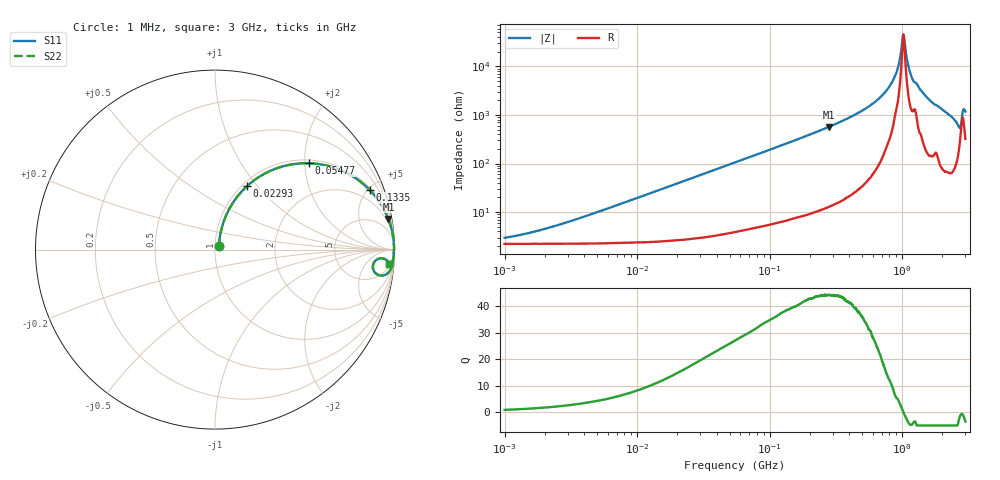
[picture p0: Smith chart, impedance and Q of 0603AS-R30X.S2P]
!s-Parameter Generated by FASTRON Sdn. Bhd.
!FASTRON P/N : 0603AS-R30X
!Keysight Technologies: E4991B_MY54100416_A.01.15
!Date created: Tue Oct 17 15:01:34 2023
!Version  : Rev01 Tue Oct 17 15:01:34 2023
!Data & Calibration Information:
!Freq	S11	S21	S12	S22
!PortZ  Port1:50+j0  Port2:50+j0
!When reading reference impedance value at option line is always used.
! Remarks : This data is being provided solely for informational purposes.
# Hz S dB R 50
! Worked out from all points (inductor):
!   1601 points, 1 MHz to 3 GHz, reference 50 ohm
!   read as one part in series: L = 309 nH near 3.459 MHz
!   highest Q = 44.3 at 278.5 MHz (marker M1), where L = 323 nH
!   self-resonance near 1.018 GHz
!   S11 on the Smith chart (normalised r, x): 1 MHz: 1.04, +0.04; 22.93 MHz: 1.05, +0.89; 54.77 MHz: 1.08, +2.10; 133.5 MHz: 1.13, +5.14; 3 GHz: 7, -23
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1000000  -30.77 40.4  -0.19 -1.1  -0.19 -1.1  -30.77 40.4
3804036  -22.45 69.0  -0.22 -4.1  -0.22 -4.1  -22.45 69.0
1.447069e7  -11.55 69.7  -0.52 -15.3  -0.52 -15.3  -11.55 69.7
2.293104e7  -8.04 63.2  -0.97 -23.3  -0.97 -23.3  -8.04 63.2
5.477226e7  -2.95 42.5  -3.39 -45.3  -3.39 -45.3  -2.95 42.5
1.334721e8  -0.69 21.1  -8.89 -67.5  -8.89 -67.5  -0.69 21.1
2.083556e8  -0.30 13.6  -12.54 -75.0  -12.54 -75.0  -0.30 13.6
2.785165e8  -0.17 10.0  -15.21 -78.7  -15.21 -78.7  -0.17 10.0
5.473095e8  -0.04 4.0  -23.15 -84.3  -23.15 -84.3  -0.04 4.0
7.925923e8  -0.02 1.5  -31.33 -83.9  -31.33 -83.9  -0.02 1.5
9.117997e8  -0.02 0.7  -37.96 -78.6  -37.96 -78.6  -0.02 0.7
9.490412e8  -0.02 0.5  -41.55 -74.7  -41.55 -74.7  -0.02 0.5
9.977393e8  -0.02 0.2  -49.43 -51.4  -49.43 -51.4  -0.02 0.2
1.023018e9  -0.02 -0.0  -53.14 2.4  -53.14 2.4  -0.02 -0.0
1.048936e9  -0.02 -0.2  -48.92 51.4  -48.92 51.4  -0.02 -0.2
1.113852e9  -0.02 -0.5  -40.17 75.1  -40.17 75.1  -0.02 -0.5
1.182785e9  -0.03 -1.0  -35.41 77.1  -35.41 77.1  -0.03 -1.0
1.526649e9  -0.04 -2.4  -27.45 83.3  -27.45 83.3  -0.04 -2.4
2.660507e9  -0.50 -8.8  -15.94 65.1  -15.94 65.1  -0.50 -8.8
2.727913e9  -0.90 -8.2  -15.48 50.0  -15.48 50.0  -0.90 -8.2
2.911267e9  -0.37 -3.5  -22.70 54.0  -22.70 54.0  -0.37 -3.5
3e9  -0.23 -4.6  -21.60 69.5  -21.60 69.5  -0.23 -4.6
